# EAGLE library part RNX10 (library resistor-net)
RESISTOR NETWORK
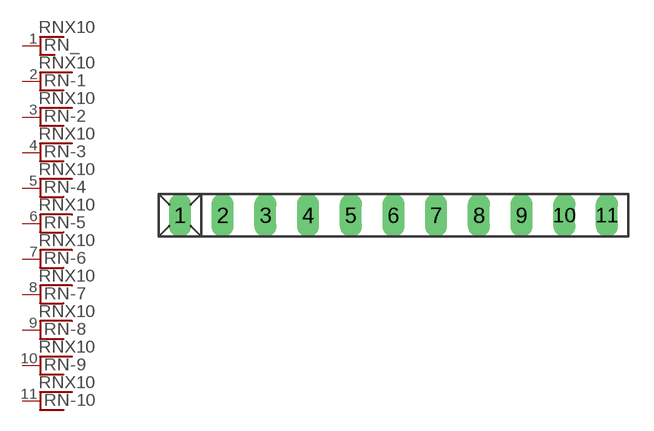
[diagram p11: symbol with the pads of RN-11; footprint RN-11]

Designator prefix RN; gates -1=RNX -2=RNX -3=RNX -4=RNX -5=RNX -6=RNX -7=RNX -8=RNX -9=RNX -10=RNX _=RN_1

## RNX10 (OC_FARNELL: unknown; OC_NEWARK: unknown)  [RN-11]
1  _:1  pas
2  -1:1  pas
3  -2:1  pas
4  -3:1  pas
5  -4:1  pas
6  -5:1  pas
7  -6:1  pas
8  -7:1  pas
9  -8:1  pas
10  -9:1  pas
11  -10:1  pas

## Footprint RN-11 (pad centres in mm)
RESISTOR NETWORK
drill 0.813 long: 1 -12.7,0; 2 -10.16,0; 3 -7.62,0; 4 -5.08,0; 5 -2.54,0; 6 0,0; 7 2.54,0; 8 5.08,0; 9 7.62,0; 10 10.16,0; 11 12.7,0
